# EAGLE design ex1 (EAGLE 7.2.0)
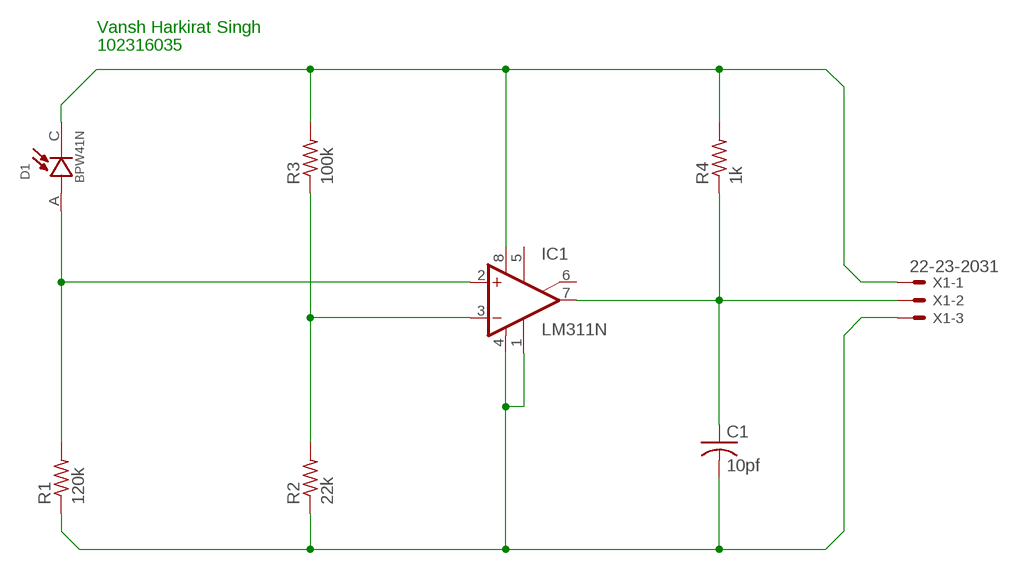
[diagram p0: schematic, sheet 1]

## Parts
C1  10pf  C-US025-024X044  [C025-024X044]
D1  BPW41N  [DIO_BPW41N]
IC1  LM311N  [DIL08]
R1  120k  R-US_0204/5  [0204/5]
R2  22k  R-US_0204/5  [0204/5]
R3  100k  R-US_0204/5  [0204/5]
R4  1k  R-US_0204/5  [0204/5]
X1  22-23-2031  [22-23-2031]

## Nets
N$1: D1.C IC1.8(V+) R3.2 R4.2 X1.1
N$2: D1.A IC1.2(+IN) R1.2
N$3: IC1.3(-IN) R2.2 R3.1
N$4: C1.2 IC1.1(GND) IC1.4(V-) R1.1 R2.1 X1.3
N$7: C1.1 IC1.7(OUT) R4.1 X1.2
Unconnected: IC1.5(ON) IC1.6(ON/STR)

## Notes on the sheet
- Vansh Harkirat Singh
- 102316035

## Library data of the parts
C1 = rcl:C-US: CAPACITOR, American symbol
D1 = BPW41N:BPW41N: BPW41N Series 65° Side View 950 nm PIN Photodiode Check availability; AVAILABILITY: In Stock; DESCRIPTION: Photodiode 940nm 130° Radial, Side View; MF: Vishay Semiconductor Opto Division; MP: BPW41N; PACKAGE: None; PRICE: None; PURCHASE-URL: https://pricing.snapeda.com/search/part/BPW41N/?ref=eda
IC1 = linear:LM311: COMPARATOR
R1-R4 = rcl:R-US_: RESISTOR, American symbol
X1 = con-molex:22-23-2031: .100" (2.54mm) Center Header - 3 Pin; MF: MOLEX; MPN: 22-23-2031; OC_FARNELL: 1462950; OC_NEWARK: 30C0862

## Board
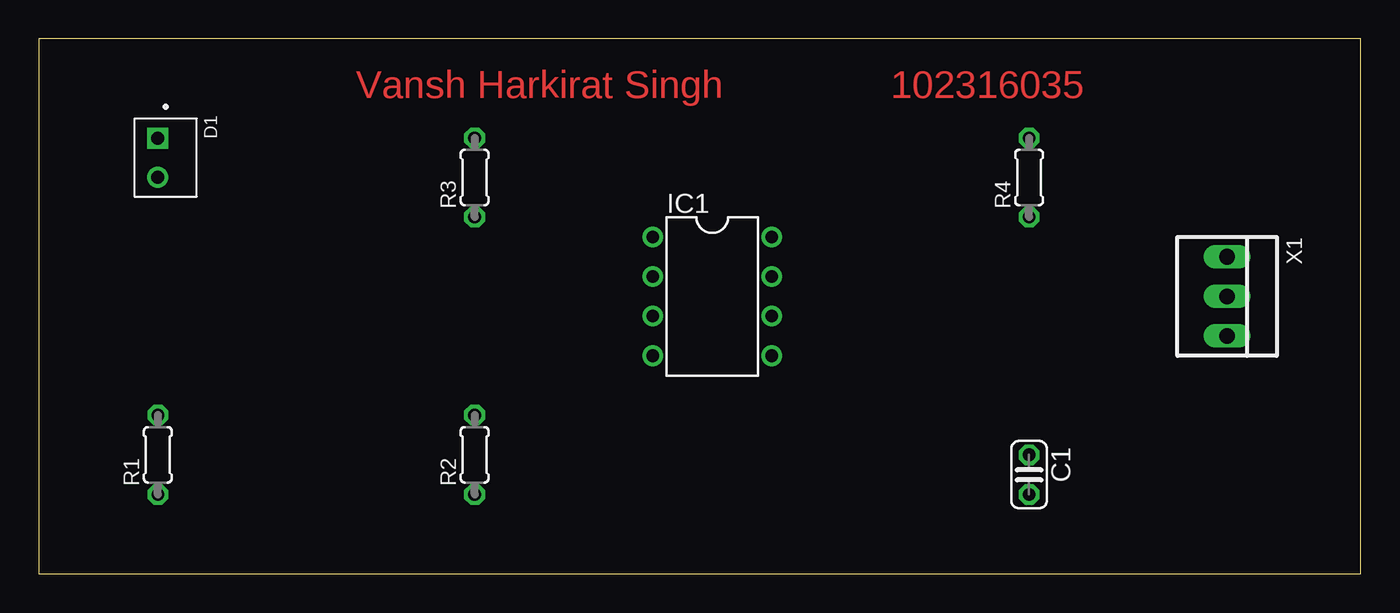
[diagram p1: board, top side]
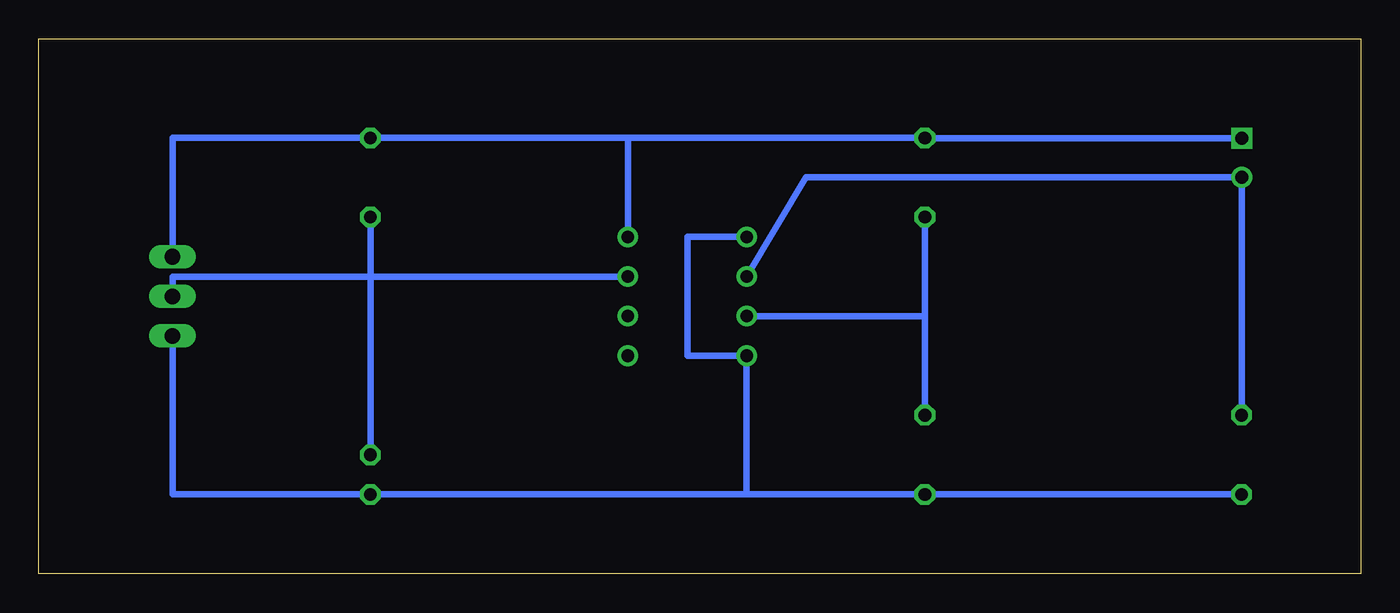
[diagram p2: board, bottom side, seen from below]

Size 84.76 x 34.28 mm. Coordinates in mm from the lower left corner, seen from the top.
Outline: 0,0 84.76,0 84.76,34.28 0,34.28 0,0
Copper layers (1*16): Top 0.035mm / dielectric 1.5mm / Bottom 0.035mm
Design rules "default": minimum track width 10mil, minimum drill 24mil, track to track 8mil, track to pad 8mil, pad to pad 8mil, via to via 8mil, smd to smd 8mil, copper to edge 40mil, drill to drill 8mil, minimum pad ring 10mil, minimum via ring 8mil, stop-mask expansion 4mil, vias tented up to drill 0mil, thermal gap 10mil

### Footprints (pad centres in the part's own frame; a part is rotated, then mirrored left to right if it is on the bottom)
C025-024X044 = drill 0.813 octagon: 1 -1.27,0; 2 1.27,0
DIO_BPW41N = drill 0.83 pad 1.25: A 1.25,0 | drill 0.83 pad 1.25 square: C -1.25,0
DIL08 = drill 0.813 pad 1.27: 1 -3.81,-3.81; 2 -1.27,-3.81; 3 1.27,-3.81; 4 3.81,-3.81; 5 3.81,3.81; 6 1.27,3.81; 7 -1.27,3.81; 8 -3.81,3.81
0204/5 = drill 0.813 octagon: 1 -2.54,0; 2 2.54,0
22-23-2031 = drill 1 long: 1 -2.54,0; 2 0,0; 3 2.54,0

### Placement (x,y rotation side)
C1  63.5,6.35 270 top
D1  7.62,26.67 270 top
IC1  43.18,17.78 270 top
R1  7.62,7.62 90 top
R2  27.94,7.62 90 top
R3  27.94,25.4 90 top
R4  63.5,25.4 90 top
X1  76.2,17.78 270 top

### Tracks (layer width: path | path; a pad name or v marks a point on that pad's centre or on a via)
N$1
  Bottom 0.406: D1.C 27.94,27.92 R3.2 46.99,27.94 | 46.99,27.94 R4.2 76.2,27.94 X1.1 | IC1.8 46.99,27.94
N$2
  Bottom 0.406: R1.2 D1.A 35.56,25.42 IC1.2
N$3
  Bottom 0.406: R3.1 27.94,16.51 | 27.94,16.51 R2.2 | IC1.3 27.94,16.51
N$4
  Bottom 0.406: R1.1 R2.1 39.37,5.08 | X1.3 76.2,5.08 C1.2 39.37,5.08 | IC1.1 43.18,21.59 43.18,13.97 IC1.4 39.37,5.08
N$7
  Bottom 0.406: IC1.7 63.5,19.05 | 63.5,19.05 76.2,19.05 X1.2 | R4.1 63.5,19.05 | C1.1 63.5,19.05

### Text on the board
Top: Vansh Harkirat Singh | 102316035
